PROGRAM MAIN

VAR CONSTANT	
    cInitSource			: ST_MA_MultiArray_InitPars 
							:= ( eTypeCode := eMA_TypeCode_LREAL, nDims := 1, aDimSizes := [cBufferLength]);	
END_VAR

VAR
	nInputSelection		: UDINT := 1;						// Switch between hardware and function generator	
	nSample				: UDINT;
	aEl3632 AT %I*		: ARRAY[1..cOversamples] OF INT;	// Input from hardware e.g. EL3632

	aBufferSignal1				: ARRAY[1..cOversamples] OF LREAL;  // signal part 1 
	aBufferSignal2				: ARRAY[1..cOversamples] OF LREAL;  // signal part 2
	aBuffer						: ARRAY[1..cOversamples] OF LREAL;  // aBufferSignal1 + aBufferSignal2
					
	fbSource			: FB_CMA_Source :=(	stInitPars := cInitSource, 
											nOwnID := eID_Source, 
											aDestIDs := [eID_Spectrum]);	// Initialize source buffers
	fbSink				: FB_CMA_Sink := (nOwnID := eID_Sink);
	
	fbFunctionGenerator1	: FB_FunctionGenerator;	// Signal Generator
	fSetFrequency1		: LREAL := 200;		        // Hz
	fSetAmplitude1		: LREAL := 2.6;		        // peak amplitude of sin signal
	fbFunctionGenerator2	: FB_FunctionGenerator;	// Signal Generator
	fSetFrequency2		: LREAL := 1000;			// Hz
	fSetAmplitude2		: LREAL := 3.8;				// peak amplitude of sin signal	
	
	aSpectrumResult		: ARRAY[1..cFFTResult] OF LREAL;	// Copy of result
	nCountResults		: ULINT;
	
	bCalculate			: BOOL;
	(* RMS value calculation *)
	nChannel			: UDINT;
	fSum				: LREAL;
	fRmsValue			: LREAL;	
	(* max amplitude calculation *)
	fMaxAmpl			: LREAL;
	nIdxOfMaxAmpl		: UDINT;		 // index of max amplitude in spectrum result array 
	(* frequency calculation *)
	fSampleTaskCycleTime: LREAL := 1; 	// ms
	fSampleRate			: LREAL; 		// Hz  ( sample rate = oversampling factor / cycle time )
	fResolution			: LREAL; 		// Hz/Idx
	fFrequency			: LREAL; 		// Hz	
	
	fbErrHist			: FB_HRErrHist; // error monitoring
END_VAR

CASE nInputSelection OF
	0:  (* input from EL3632 *)
		FOR nSample := 1 TO cOversamples DO
			aBuffer[nSample] := INT_TO_LREAL(aEl3632[nSample]);
		END_FOR
	1:  (* signal generator *)		
		fbFunctionGenerator1(	fFrequency 	:= fSetFrequency1,
								fAmplitude 	:= fSetAmplitude1,
								eFunction 	:= E_FunctionType.Sine,
								aSignal		:= aBufferSignal1 );
		fbFunctionGenerator2(	fFrequency 	:= fSetFrequency2,
								fAmplitude 	:= fSetAmplitude2,
								eFunction 	:= E_FunctionType.Sine,
								aSignal		:= aBufferSignal2 );
		FOR nSample := 1 TO cOversamples DO
			aBuffer[nSample] := aBufferSignal1[nSample]+aBufferSignal2[nSample];
		END_FOR
END_CASE					

// Call source to collect data
fbSource.Input1D( pDataIn 			:= ADR(aBuffer),
				  nDataInSize 		:= SIZEOF(aBuffer), 
				  eElementType 		:= eMA_TypeCode_LREAL,
				  nWorkDim 			:= 0,
				  pStartIndex		:= 0,
				  nOptionPars		:= cCMA_Option_MarkInterruption ); 
IF fbSource.bError THEN
	fbErrHist.AddError(bErr:=TRUE, hrErrCode:=fbSource.hrErrorCode, sErrSource:='MAIN.fbSource'); // error monitoring
	// ToDo: if error
END_IF

// Push results to sink
fbSink.Output1D(	pDataOut 		:= ADR(aSpectrumResult), 
					nDataOutSize 	:= SIZEOF(aSpectrumResult), 
					eElementType 	:= eMA_TypeCode_LREAL, 
					nWorkDim 		:= 0,
					nElements		:= 0,
					pStartIndex 	:= 0,
					nOptionPars		:= 0,
					bNewResult		=> bCalculate );
IF fbSink.bError THEN
	fbErrHist.AddError(bErr:=TRUE, hrErrCode:=fbSink.hrErrorCode, sErrSource:='MAIN.fbSink'); // error monitoring
	// ToDo: if error
END_IF
IF bCalculate THEN
	nCountResults := fbSink.nCntResults;
	IF NOT LrealIsNaN(aSpectrumResult[1]) THEN
		// Calculate RMS value of signal
		fSum := 0;	
		FOR nChannel := 1 TO cFFTResult DO
			fSum := fSum + (aSpectrumResult[nChannel] * aSpectrumResult[nChannel]);
		END_FOR
		fRmsValue := SQRT(fSum);
		
		// Calculate max amplitude in spectrum
		fMaxAmpl := 0;
		FOR nChannel:=1 TO cFFTResult DO
			IF aSpectrumResult[nChannel] > fMaxAmpl THEN
				fMaxAmpl := aSpectrumResult[nChannel];
				nIdxOfMaxAmpl := nChannel;
			END_IF
		END_FOR
		// Calculate frequency for max amplitude [ frequency = index * (sample rate / FFT length) ]
		fSampleRate := cOversamples * (1000.0 / fSampleTaskCycleTime);
		fResolution := fSampleRate / cFFTLength;
		fFrequency := (nIdxOfMaxAmpl-1) * fResolution; // -1 to consider DC = 0*fResolution
	END_IF
	// ToDo: if new result is ready
END_IF

END_PROGRAM
